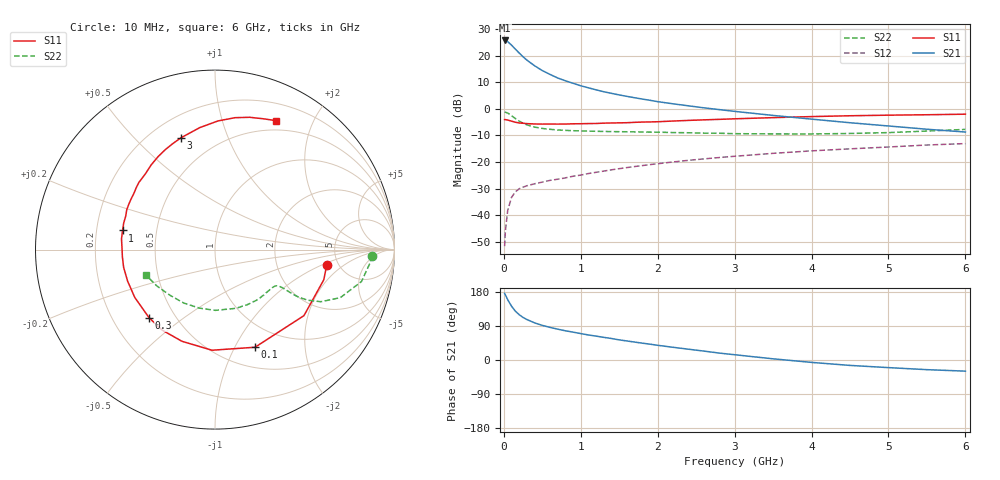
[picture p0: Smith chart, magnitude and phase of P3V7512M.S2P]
! SIEMENS Small Signal Semiconductors
! BFP181
! Si NPN RF Bipolar Junction Transistor in SOT143
! VCE = 0.75 V  IC = 12 mA
! Common Emitter S-Parameters:  March  1996
# GHz  S  MA  R  50
!  f  S11  S21  S12  S22
! GHz  MAG  ANG  MAG  ANG  MAG  ANG  MAG  ANG
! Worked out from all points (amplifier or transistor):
!   36 points, 10 MHz to 6 GHz, reference 50 ohm
!   highest |S21| = 25.8 dB at 10 MHz (marker M1)
!   |S21| within 3 dB of that: start of sweep to 140.8 MHz
!   unconditionally stable (mu >= 1): start of sweep to 15.56 MHz; 354.6 MHz to end of sweep
!   at 250 MHz: K = 0.77, MSG = 24.5 dB, |S12| = -29.5 dB
!   at 1.4 GHz: K = 2.04, MAG = 8.6 dB, |S12| = -22.9 dB
!   at 6 GHz: K = 1.86, MAG = -3.2 dB, |S12| = -13.1 dB
!   S11 on the Smith chart (normalised r, x): 10 MHz: 4.05, -1.13; 100 MHz: 0.73, -1.21; 300 MHz: 0.36, -0.38; 1 GHz: 0.31, +0.09; 3 GHz: 0.32, +0.69; 6 GHz: 0.39, +1.51
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0.01  0.6288 -7.7  19.46 175.8  0.0026 81.4  0.8756 -2.3
0.02  0.6291 -15.5  19.41 171.8  0.005 79.3  0.8667 -5.0
0.05  0.6172 -36.6  18.51 159.2  0.0122 73.8  0.8354 -12.3
0.1  0.588 -67.7  15.89 142.0  0.0216 59.9  0.7476 -21.0
0.15  0.5609 -91.7  13.34 128.9  0.0274 50.8  0.6575 -26.2
0.2  0.543 -109.8  11.28 119.5  0.0314 46.2  0.5888 -28.6
0.25  0.5365 -123.2  9.578 112.2  0.0336 42.9  0.5384 -29.6
0.3  0.5283 -134.0  8.288 106.8  0.0357 41.2  0.5008 -29.8
0.4  0.5204 -149.2  6.49 97.9  0.0389 40.3  0.454 -29.6
0.5  0.5177 -160.1  5.272 91.4  0.0418 40.1  0.4285 -29.5
0.6  0.5186 -169.0  4.464 86.0  0.0451 41.2  0.4127 -29.7
0.7  0.5176 -175.6  3.821 81.4  0.0474 42.7  0.4008 -30.2
0.8  0.5185 178.6  3.387 77.1  0.0502 43.2  0.3943 -30.8
1  0.5259 168.3  2.727 69.7  0.0567 45.1  0.3848 -33.1
1.1  0.5297 163.8  2.494 66.0  0.0607 45.5  0.3814 -34.4
1.5  0.5462 148.7  1.834 53.1  0.0749 46.8  0.3722 -40.9
2.2  0.5909 127.0  1.247 33.5  0.1002 45.1  0.3588 -55.4
3  0.651 107.0  0.899 13.9  0.1282 40.1  0.3416 -75.1
3.5  0.685 97.1  0.754 3.1  0.1456 36.4  0.3385 -89.7
4.5  0.7433 81.4  0.549 -14.3  0.177 27.8  0.3449 -120.4
5.5  0.7765 69.9  0.414 -25.5  0.2089 19.5  0.3826 -148.3
6  0.7952 64.6  0.367 -29.4  0.2224 14.7  0.4113 -160.2
